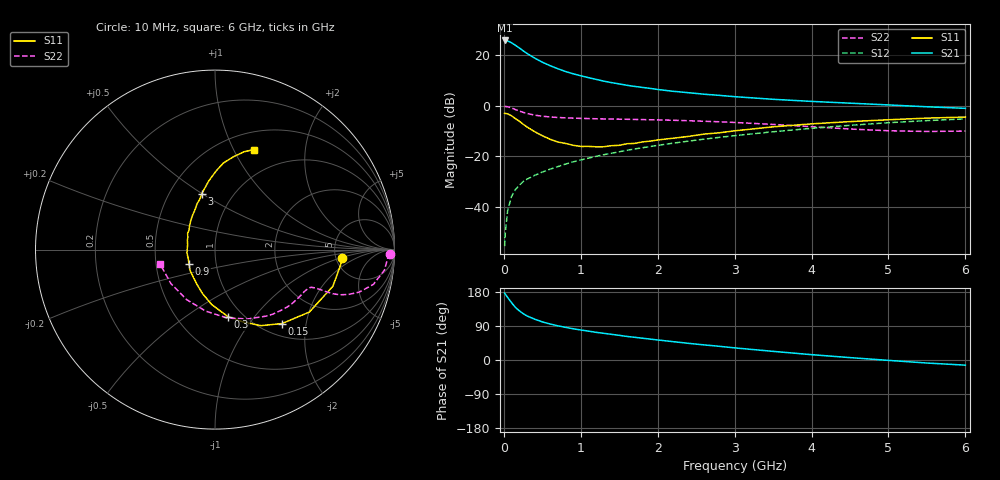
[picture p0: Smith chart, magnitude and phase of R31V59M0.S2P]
! SIEMENS Small Signal Semiconductors
! BFR181
! Si NPN RF Bipolar Junction Transistor in SOT23
! VCE = 1.5 V  IC = 9 mA
! Common Emitter S-Parameters:  May  1996
# GHz  S  MA  R  50
!  f  S11  S21  S12  S22
! GHz  MAG  ANG  MAG  ANG  MAG  ANG  MAG  ANG
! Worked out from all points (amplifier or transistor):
!   36 points, 10 MHz to 6 GHz, reference 50 ohm
!   highest |S21| = 25.7 dB at 10 MHz (marker M1)
!   |S21| within 3 dB of that: start of sweep to 203 MHz
!   unconditionally stable (mu >= 1): 613.1 MHz to 2.883 GHz
!   at 250 MHz: K = 0.64, MSG = 25.8 dB, |S12| = -30.0 dB
!   at 1.4 GHz: K = 1.12, MAG = 11.8 dB, |S12| = -18.8 dB
!   at 6 GHz: K = 0.88, MSG = 2.1 dB, |S12| = -5.2 dB
!   S11 on the Smith chart (normalised r, x): 10 MHz: 5.70, -1.05; 150 MHz: 1.23, -1.47; 300 MHz: 0.86, -0.75; 900 MHz: 0.74, -0.12; 3 GHz: 0.72, +0.50; 6 GHz: 0.69, +1.20
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0.01  0.7102 -3.7  19.3 176.9  0.0017 88.9  0.9725 -1.3
0.02  0.7044 -7.3  19.26 173.6  0.0033 84.6  0.9636 -2.8
0.05  0.6877 -17.3  18.88 164.8  0.0086 81.4  0.951 -6.9
0.1  0.6304 -33.5  17.37 151.3  0.0163 74.8  0.9034 -12.4
0.15  0.5561 -47.8  15.53 138.7  0.0221 69.5  0.8384 -16.4
0.2  0.4949 -58.9  13.77 130.1  0.0269 67.1  0.7841 -18.6
0.25  0.4321 -68.8  12.11 122.5  0.0318 64.8  0.7398 -19.9
0.3  0.3813 -78.9  10.74 116.4  0.0354 65.4  0.7025 -20.5
0.4  0.3073 -93.3  8.683 107.8  0.0423 65.2  0.6512 -20.8
0.5  0.256 -105.5  7.193 100.6  0.0491 65.7  0.6194 -20.8
0.6  0.2183 -117.4  6.153 95.1  0.0559 66.5  0.5991 -20.9
0.7  0.1925 -130.0  5.361 90.3  0.0628 67.6  0.585 -21.2
0.9  0.1658 -150.4  4.259 82.5  0.078 68.3  0.5676 -22.0
1.1  0.1574 -173.4  3.569 76.2  0.0925 69.1  0.5567 -23.7
1.3  0.155 169.7  3.044 70.4  0.1081 68.9  0.5486 -25.6
1.6  0.1777 149.0  2.521 62.2  0.1317 68.3  0.5391 -29.1
2.2  0.2282 123.3  1.921 48.4  0.1823 65.4  0.5156 -37.9
3  0.3193 103.4  1.505 32.0  0.2563 59.4  0.4668 -52.6
3.5  0.3825 95.4  1.336 22.8  0.3061 54.6  0.427 -64.9
4.5  0.4852 84.4  1.12 6.3  0.41 42.9  0.3465 -98.7
5.5  0.5684 73.5  0.951 -8.0  0.5078 29.0  0.3101 -142.6
6  0.597 68.9  0.886 -13.6  0.549 21.5  0.3155 -164.9
